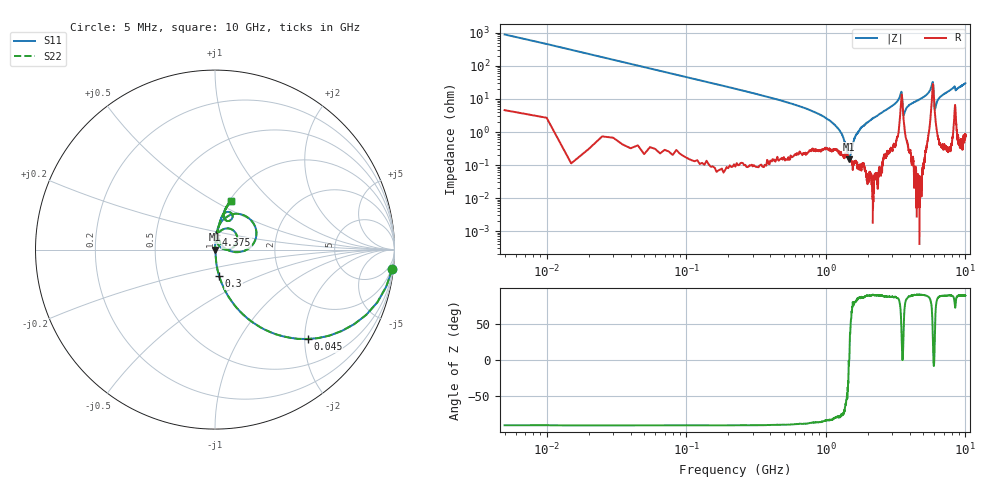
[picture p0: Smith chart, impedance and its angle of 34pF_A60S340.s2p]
! Amotech Co.,Ltd.
! http://www.amotech.co.kr/
! Part Number: A60S340
! These Parameters are Measured in Series Mode Connection
! Operation Temp=25[degC], DC Bias Voltage=0[V]
! Freq. Start=5[MHz] Stop=10[GHz], 2000[Steps]
! Date: Monday, July 13, 2020, 01:41:52
# GHZ S RI R 50.000000
!Freq.(Hz) S11(Real) S11(Imag) S21(Real) S21(Imag) S12(Real) S12(Imag) S22(Real) S22(Imag)
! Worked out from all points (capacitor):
!   2000 points, 5 MHz to 10 GHz, reference 50 ohm
!   read as one part in series: C = 34.2 pF near 55 MHz
!   lowest |Z| = 152 mohm at 1.475 GHz (marker M1)
!   series resonance near 1.47 GHz, so ESL is about 340 pH
!   S11 on the Smith chart (normalised r, x): 5 MHz: 1, -18; 45 MHz: 1.01, -2.06; 300 MHz: 1.00, -0.30; 4.375 GHz: 1.00, +0.16; 10 GHz: 1.02, +0.61
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0.005  0.9871 -0.1101  0.0129 0.1101  0.0129 0.1101  0.9871 -0.1101
0.045  0.5156 -0.4978  0.4844 0.4978  0.4844 0.4978  0.5156 -0.4978
0.075  0.2774 -0.4457  0.7226 0.4457  0.7226 0.4457  0.2774 -0.4457
0.125  0.1218 -0.3256  0.8782 0.3256  0.8782 0.3256  0.1218 -0.3256
0.3  0.0231 -0.1473  0.9769 0.1473  0.9769 0.1473  0.0231 -0.1473
1.17  0.00321 -0.0154  0.9968 0.0154  0.9968 0.0154  0.00321 -0.0154
1.3  0.00207 -0.0084  0.9979 0.0084  0.9979 0.0084  0.00207 -0.0084
1.475  0.00151 2.68e-05  0.9985 -2.68e-05  0.9985 -2.68e-05  0.00151 2.68e-05
1.675  0.00131 0.00892  0.9987 -0.00892  0.9987 -0.00892  0.00131 0.00892
2.15  0.000768 0.0252  0.9992 -0.0252  0.9992 -0.0252  0.000768 0.0252
3.34  0.0219 0.0965  0.9781 -0.0965  0.9781 -0.0965  0.0219 0.0965
3.475  0.1127 0.0957  0.8873 -0.0957  0.8873 -0.0957  0.1127 0.0957
3.625  0.0197 0.0258  0.9803 -0.0258  0.9803 -0.0258  0.0197 0.0258
3.845  0.00778 0.0574  0.9922 -0.0574  0.9922 -0.0574  0.00778 0.0574
4.375  0.00742 0.0815  0.9926 -0.0815  0.9926 -0.0815  0.00742 0.0815
5.005  0.0137 0.1128  0.9863 -0.1128  0.9863 -0.1128  0.0137 0.1128
5.815  0.2085 0.1543  0.7915 -0.1543  0.7915 -0.1543  0.2085 0.1543
6.055  0.0352 0.0297  0.9648 -0.0297  0.9648 -0.0297  0.0352 0.0297
6.67  0.018 0.1174  0.982 -0.1174  0.982 -0.1174  0.018 0.1174
8.335  0.0788 0.2098  0.9212 -0.2098  0.9212 -0.2098  0.0788 0.2098
8.53  0.0614 0.1635  0.9386 -0.1635  0.9386 -0.1635  0.0614 0.1635
10  0.0898 0.2734  0.9102 -0.2734  0.9102 -0.2734  0.0898 0.2734
